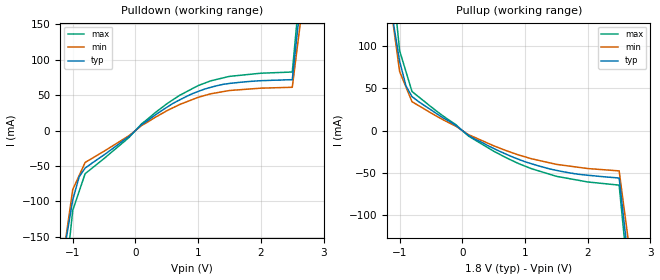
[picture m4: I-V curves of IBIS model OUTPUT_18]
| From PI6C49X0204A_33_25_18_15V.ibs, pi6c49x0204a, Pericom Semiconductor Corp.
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|   Model OUTPUT_18
[Model] OUTPUT_18
Model_type Output
Vref = 0.0000V
Rref = 50ohms
Vmeas = 0.90V
| variable   typ   min   max
C_comp   2.000pF   1.8pF	2.2pF
[Voltage Range]   1.8   1.7   1.9
[POWER Clamp Reference]   1.800V   NA   NA
[GND Clamp Reference]   0.000V   0	 0
[Pullup Reference]   1.8   1.7   1.9
[Pulldown Reference]   0.000V   NA   NA
[Temperature Range]   25.00   85.00   -45.000
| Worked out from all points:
|   slope of the pulldown table from 0 to 0.27 V, typ, clamps not added: 14.2 ohm
|   slope of the pullup table from 0 to 0.27 V, typ, clamps not added: 21.6 ohm
[Pulldown]
| Voltage   I(typ)   I(min)  I(max)
-1.8V     -917.2mA   -779.6mA   -1.055A
-1.1V     -151.1mA   NA         NA
-999.3mV  -97.83mA   -83.16mA   -112.5mA
-898.2mV  -65.44mA   NA         NA
-802mV    -52.94mA   -45mA      -60.88mA
99.45mV   8.25mA     7.012mA    9.487mA
498.6mV   32.62mA    27.73mA    37.51mA
898.2mV   51.61mA    NA         NA
1.202V    60.91mA    51.77mA    70.05mA
1.5V      66.36mA    56.41mA    76.31mA
2.501V    71.7mA     60.94mA    82.46mA
3.099V    566.4mA    481.4mA    651.3mA
[Pullup]   |Note: Vtable = Vcc - Voutput
| Voltage   I(typ)   I(min)   I(max)
-1.8V     845.1mA    718.3mA    971.9mA
-1.1V     128.3mA    NA         NA
-999.4mV  82.22mA    69.89mA    94.55mA
-898.2mV  52.83mA    NA         NA
-802mV    40.18mA    34.15mA    46.21mA
-99.45mV  5.88mA     4.998mA    6.762mA
99.44mV   -5.76mA    -4.896mA   -6.624mA
700.9mV   -28.06mA   -23.85mA   -32.27mA
1.1V      -39.25mA   -33.36mA   -45.14mA
1.798V    -51.22mA   NA         NA
2.501V    -56.24mA   -47.8mA    -64.68mA
3.197V    -517.9mA   -440.2mA   -595.6mA
[Ramp]
| variable   typ   min   max
dV/dt_r   1.8V/941.0p   1.8V/1041.0p   1.8V/841.0p
dV/dt_f   1.8V/806.0p   1.8V/1006.0p   1.8V/706.0p
R_load = 50ohms
